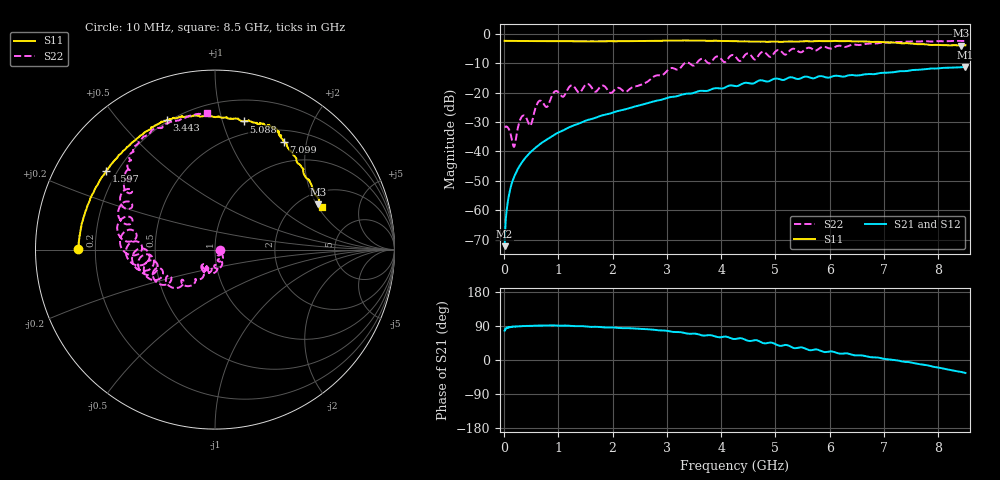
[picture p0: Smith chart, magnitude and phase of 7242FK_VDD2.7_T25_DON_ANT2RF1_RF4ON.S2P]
!Agilent Technologies,E5071C,MY46417908,A.11.23
!Date: Wed Dec 09 15:39:53 2020
!Data & Calibration Information:
!Freq	S11:SOLT2(ON)	S21:SOLT2(ON)	S12:SOLT2(ON)	S22:SOLT2(ON)
!PortZ  Port1:50+j0  Port2:50+j0
!Above PortZ is port z conversion or system Z0 setting when saving the data.
!When reading, reference impedance value at option line is always used.
# Hz S dB R 50
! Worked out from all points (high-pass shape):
!   1601 points, 10 MHz to 8.5 GHz, reference 50 ohm
!   highest |S21| = -11.29 dB at 8.5 GHz (marker M1); lowest = -72.2 dB at 10 MHz (marker M2)
!   |S21| within 3 dB of the highest: 6.084 GHz to 6.161 GHz (77.48 MHz wide, 1.27 % of centre); 6.31 GHz to end of sweep
!   lowest |S11| = -4.0 dB at 8.42 GHz (marker M3), VSWR 4.38, Z = 124 + j104 ohm
!   |S11| at or under -10 dB: nowhere
!   |S22| runs from -38.4 to -2.4 dB; largest |S21 - S12| = 0.0032
!   S11 on the Smith chart (normalised r, x): 10 MHz: 0.13, +0.00; 1.597 GHz: 0.16, +0.32; 3.443 GHz: 0.19, +0.68; 5.088 GHz: 0.38, +1.17; 7.099 GHz: 0.66, +1.62; 8.5 GHz: 2.68, +2.15
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1e7  -2.34 179.8  -72.21 77.3  -72.11 74.9  -31.70 -3.0
8.42875e7  -2.38 178.2  -55.40 85.9  -55.27 86.6  -32.23 -34.4
1.851062e8  -2.40 176.1  -48.66 88.0  -48.69 88.3  -38.44 -24.1
3.230688e8  -2.41 173.1  -43.84 89.2  -43.88 89.3  -28.22 -30.3
4.875625e8  -2.43 169.6  -40.24 89.8  -40.24 90.1  -31.22 -49.8
6.308312e8  -2.45 166.6  -37.96 90.7  -37.96 90.9  -23.10 -52.8
7.900188e8  -2.48 163.2  -35.90 91.0  -35.92 91.0  -24.85 -67.9
9.439e8  -2.50 159.6  -34.13 91.1  -34.14 91.3  -19.48 -77.4
1.246356e9  -2.51 152.4  -31.37 89.9  -31.39 89.9  -17.50 -98.5
1.426769e9  -2.52 148.3  -30.11 89.4  -30.11 89.4  -19.31 -99.6
1.596569e9  -2.53 144.1  -29.03 87.3  -29.03 87.3  -17.81 -123.2
2.243931e9  -2.48 130.0  -25.60 84.3  -25.61 84.3  -19.69 -119.1
2.843538e9  -2.36 118.7  -22.59 78.4  -22.60 78.4  -14.08 -123.3
3.443144e9  -2.28 110.4  -20.30 69.1  -20.30 69.1  -10.39 -151.0
4.255e9  -2.48 97.0  -17.74 55.4  -17.75 55.4  -7.59 -174.2
4.695419e9  -2.62 88.1  -15.89 50.0  -15.90 50.0  -7.13 -168.4
5.088081e9  -2.72 77.5  -15.49 37.4  -15.46 37.3  -5.69 169.8
5.671769e9  -2.56 67.2  -15.06 26.0  -15.01 26.0  -5.03 151.4
7.088538e9  -2.92 57.6  -13.13 1.4  -13.18 1.3  -2.96 129.7
7.09915e9  -2.94 57.5  -13.12 1.2  -13.18 1.2  -2.95 129.7
8.420406e9  -4.03 23.6  -11.35 -31.4  -11.40 -31.5  -2.42 95.3
8.5e9  -3.87 21.7  -11.29 -34.2  -11.37 -34.1  -2.36 93.3
